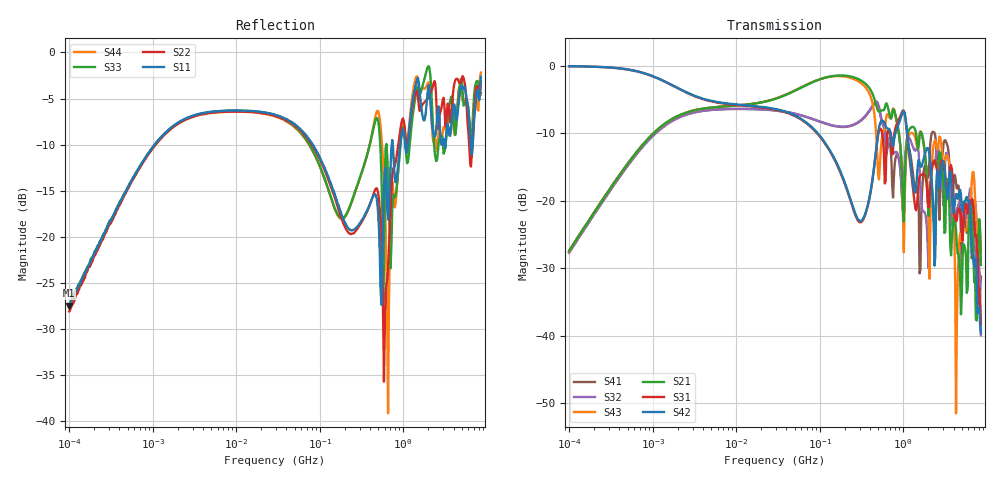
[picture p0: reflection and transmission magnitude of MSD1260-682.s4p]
# MHz S MA R 50
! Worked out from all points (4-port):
!   498 points, 100 kHz to 8.5 GHz, reference 50 ohm
!   strongest paths, dB at 100 kHz, 1.698 MHz, 29.49 MHz, 500.7 MHz, 8.5 GHz:
!     S42: -0.1, -2.9, -6.4, -9.9, -39.6
!     S31: -0.1, -2.9, -6.5, -10.3, -38.2
!     S21: -27.4, -7.9, -4.9, -6.7, -29.5
!     S43: -27.5, -7.9, -4.9, -16.0, -27.6
!     S32: -27.7, -8.2, -6.6, -5.7, -39.9
!     S41: -27.7, -8.2, -6.6, -5.9, -31.2
!   lowest |S11| = -27.5 dB at 100 kHz (marker M1), VSWR 1.09, Z = 50.3 + j4.22 ohm
!   |S11| at or under -10 dB: 82.48 MHz to 729 MHz (646.5 MHz wide, 159 % of centre); 748.1 MHz to 920 MHz (171.9 MHz wide, 20.6 % of centre); 6.412 GHz to 6.784 GHz (371.6 MHz wide, 5.63 % of centre)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
0.1  0.0421 83.8  0.04255 83.4  0.9897 -2.5  0.0413 -97.3
     0.04255 83.4  0.03917 84.8  0.04104 -96.9  0.9915 -2.4
     0.9897 -2.5  0.04104 -96.9  0.04124 84.5  0.04214 83.1
     0.0413 -97.3  0.9915 -2.4  0.04214 83.1  0.04215 85.2
121.5084  0.221 -57.1  0.8211 -10.8  0.2532 -89.3  0.3693 84.1
          0.8211 -10.8  0.2146 -59.8  0.3712 82.8  0.2568 -88.7
          0.2532 -89.3  0.3712 82.8  0.1918 -51.5  0.8203 -13.5
          0.3693 84.1  0.2568 -88.7  0.8203 -13.5  0.1899 -49.8
467.5077  0.1684 -50.6  0.5281 -93.2  0.2222 62.1  0.5341 -34.5
          0.5281 -93.2  0.1818 -56.1  0.5426 -34.6  0.2238 69.3
          0.2222 62.1  0.5426 -34.6  0.4309 -59.5  0.3498 -122.9
          0.5341 -34.5  0.2238 69.3  0.3498 -122.9  0.4557 -52.5
658.5124  0.1236 -38.9  0.4848 -112.2  0.3307 -16.9  0.2666 -89.5
          0.4848 -112.2  0.06858 -3.9  0.2628 -70.6  0.3424 -38.6
          0.3307 -16.9  0.2628 -70.6  0.2095 -112.9  0.4332 -88.2
          0.2666 -89.5  0.3424 -38.6  0.4332 -88.2  0.01096 64.3
1970.81  0.6264 -158.2  0.09732 86.9  0.09875 176.0  0.1476 -163.2
         0.09732 86.9  0.5631 -160.4  0.04242 152.1  0.2451 159.7
         0.09875 176.0  0.04242 152.1  0.8363 -170.4  0.105 90.7
         0.1476 -163.2  0.2451 159.7  0.105 90.7  0.6848 -176.6
3332.473  0.3927 50.3  0.1396 -107.6  0.1282 18.2  0.2625 15.0
          0.1396 -107.6  0.4808 29.8  0.2245 19.2  0.111 17.7
          0.1282 18.2  0.2245 19.2  0.3802 43.8  0.2174 -37.2
          0.2625 15.0  0.111 17.7  0.2174 -37.2  0.4196 41.2
8500  0.7385 -31.5  0.03348 -138.5  0.01226 -132.4  0.02745 -101.0
      0.03348 -138.5  0.6967 -41.0  0.01008 37.2  0.01045 -153.6
      0.01226 -132.4  0.01008 37.2  0.6025 -41.0  0.04152 -144.9
      0.02745 -101.0  0.01045 -153.6  0.04152 -144.9  0.777 -40.1
